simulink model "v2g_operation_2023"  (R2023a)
settings: Solver=VariableStepAuto  StartTime=0.0  StopTime=0.1  FixedStep=1e-7  MaxStep=1e-5  RelTol=1e-3
libraries: spsMosfetLib x4, spsCurrentMeasurementLib x2, spsACVoltageSourceLib x1, spsPowerLib x1, spsVoltageMeasurementLib x1, spsDCVoltageSourceLib x1, spsSeriesRLCBranchLib x1, simulink x1, spspowerguiLib x1

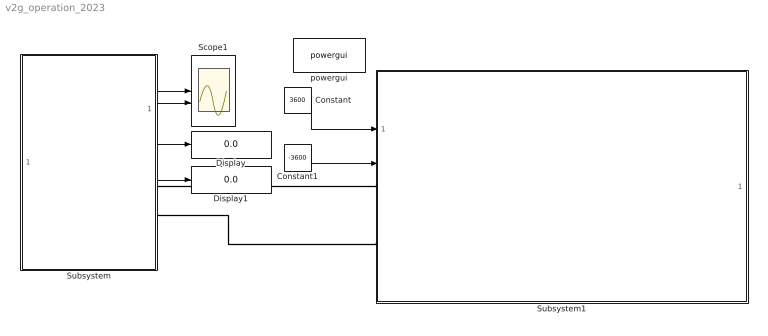
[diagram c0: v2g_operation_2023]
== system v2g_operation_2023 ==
  Constant : Constant  Value=3600
  Constant1 : Constant  Value=-3600
  Display : Display
  Display1 : Display
  Scope1 : Scope  NumInputPorts=2
  Subsystem : Subsystem
  Subsystem1 : Subsystem
  powergui : spspowerguiLib/powergui  Priority=1  SimulationMode=Continuous  SampleTime=50e-6  frequency=60  Iterations=50  frequencyindice=60  Pbase=100e6  ErrMax=1e-4  UnitsV=kV  UnitsW=MW  buscounter=0  FunctionMessages=off  echomessages=off  EnableUseOfTLC=off  CurrentSourceSwitches=off  DisableSnubberDevices=off  DisableRonSwitches=off  DisableVfSwitches=off  DisplayEquations=off  AutomaticDiscreteSolvers=off  SolverType=Tustin/Backward Euler (TBE)  Interpol=off  ExternalGateDelay=off  methode=off  Ts=100  x0status=blocks  SPID=on  SwTol=0  HookPort=off  NonlinearTolerance=1e-4  nMaxIteration=100  ContinueOnMaxIteration=off  RestoreLinks=warning  ResistiveCurrentMeasurement=off  Frange=[0:2:500]  Ylog=off  Xlog=on  ShowGrid=off  save=off  variable=ZData  structure=0  ZoomFFT=off  StartTime=0.0  cycles=1  DisplayStyle=1  fundamental=60  FreqAxis=off  MaxFrequency=1000  frequencyindicesteady=1  RmsSteady=1  display=off
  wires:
  Subsystem/1(vac) -> Scope1/1
  Subsystem/2(iac) -> Scope1/2
  Subsystem/3(P) -> Display/1
  Subsystem/4(Q) -> Display1/1
  Constant/1 -> Subsystem1/1(Pref)
  Constant1/1 -> Subsystem1/2(Qref)
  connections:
  Subsystem/RConn1 -- Subsystem1/LConn1
  Subsystem/RConn2 -- Subsystem1/LConn2

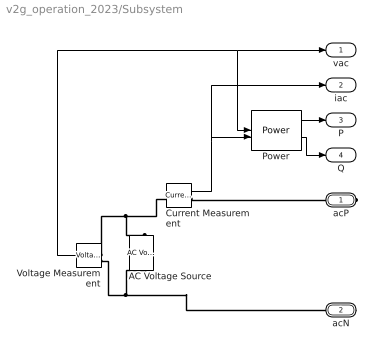
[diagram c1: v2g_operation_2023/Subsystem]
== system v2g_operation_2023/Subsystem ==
  AC Voltage Source : spsACVoltageSourceLib/AC Voltage Source  Amplitude=220*sqrt(2)  Phase=0  Frequency=60  SampleTime=0  Measurements=None  BusType=swing  Pref=10e3  Qref=0  Qmin=-inf  Qmax=+inf
  Current Measurement : spsCurrentMeasurementLib/Current Measurement  PhasorSimulation=off  OutputType=Complex  PSBequivalent=0
  Power : spsPowerLib/Power  Freq=60  Vinit=[1, 0]  Iinit=[1, 0]  Ts=0
  Voltage Measurement : spsVoltageMeasurementLib/Voltage Measurement  PhasorSimulation=off  OutputType=Complex  PSBequivalent=0
  acP : PMIOPort  Side=Right
  acN : PMIOPort  Port=2  Side=Right
  vac : Outport
  iac : Outport  Port=2
  P : Outport  Port=3
  Q : Outport  Port=4
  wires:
  Voltage Measurement/1 -> Power/1, vac/1
  Current Measurement/1 -> Power/2, iac/1
  Power/1 -> P/1
  Power/2 -> Q/1
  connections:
  Voltage Measurement/LConn2 -- acN/RConn1 -- AC Voltage Source/LConn1
  Voltage Measurement/LConn1 -- AC Voltage Source/RConn1 -- Current Measurement/LConn1
  Current Measurement/RConn1 -- acP/RConn1

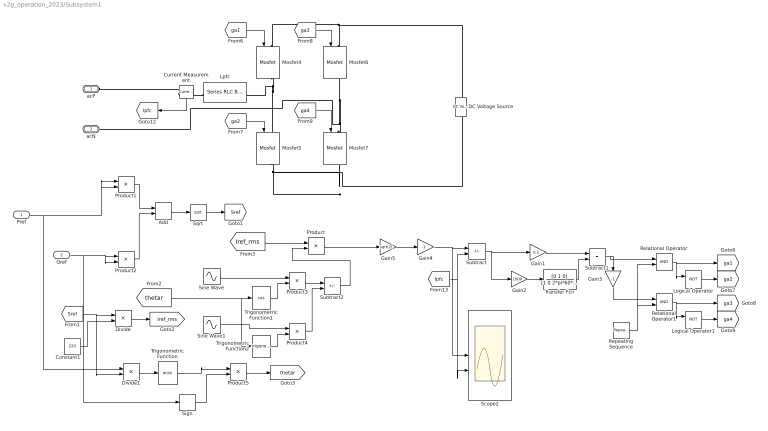
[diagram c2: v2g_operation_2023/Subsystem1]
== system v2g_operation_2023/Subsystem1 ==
  Pref : Inport
  Qref : Inport  Port=2
  Add : Sum
  Constant1 : Constant  Value=220
  Current Measurement : spsCurrentMeasurementLib/Current Measurement  PhasorSimulation=off  OutputType=Complex  PSBequivalent=0
  DC Voltage Source : spsDCVoltageSourceLib/DC Voltage Source  Amplitude=380  Measurements=None
  Divide : Product  Inputs=*/
  Divide1 : Product  Inputs=*/
  Gain1 : Gain  Gain=0.1
  Gain2 : Gain  Gain=1000
  Gain3 : Gain  Gain=-1
  Gain4 : Gain  Gain=-1
  Gain5 : Gain  Gain=sqrt(2)
  Logical Operator : Logic  Operator=NOT  AllPortsSameDT=off  OutDataTypeStr=boolean
  Logical Operator1 : Logic  Operator=NOT  AllPortsSameDT=off  OutDataTypeStr=boolean
  Lpfc : spsSeriesRLCBranchLib/Series RLC Branch  LConnTagsString=__new0  RConnTagsString=__new0  BranchType=L  Resistance=20  Inductance=5e-3  SetiL0=off  InitialCurrent=0  Capacitance=3e-3  Setx0=on  InitialVoltage=380  Measurements=Branch current
  Mosfet{4..7} (4 alike) : spsMosfetLib/Mosfet  Ron=0.1  Lon=0  Rd=0.01  Vfd=0  IC=0  Rs=1e5  Cs=inf  Measurements=on
  Product{,1..5} (6 alike) : Product
  Relational Operator : RelationalOperator  OutDataTypeStr=boolean  RndMeth=Simplest
  Relational Operator1 : RelationalOperator  OutDataTypeStr=boolean  RndMeth=Simplest
  Repeating Sequence : simulink/Sources/Repeating Sequence  rep_seq_t=[0 0.00005]  rep_seq_y=[0 1]
  Scope2 : Scope  NumInputPorts=2
  Sign : Signum
  Sine Wave : Sin  Frequency=2*pi*60  SampleTime=0
  Sine Wave1 : Sin  Frequency=2*pi*60  Phase=pi/2  SampleTime=0
  Sqrt : Sqrt
  Subtract : Sum  Inputs=+-
  Subtract1 : Sum
  Subtract2 : Sum  Inputs=+-
  Transfer Fcn : TransferFcn  Numerator=[0 1 0]  Denominator=[1 0 2*pi*60*2*pi*60]
  Trigonometric Function : Trigonometry  Operator=acos
  Trigonometric Function1 : Trigonometry  Operator=cos
  Trigonometric Function2 : Trigonometry
  acP : PMIOPort  Side=Left
  acN : PMIOPort  Port=2  Side=Left
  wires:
  Repeating Sequence/1 -> Relational Operator1/2, Relational Operator/2
  [ga2] -> Mosfet5/1
  [ga4] -> Mosfet7/1
  Subtract1/1 -> Gain3/1, Relational Operator/1
  Gain1/1 -> Subtract1/1
  [ga3] -> Mosfet6/1
  Product/1 -> Gain5/1
  [Ipfc] -> Subtract/2, Scope2/2
  Relational Operator/1 -> [ga1], Logical Operator/1
  Subtract/1 -> Gain2/1, Gain1/1
  Relational Operator1/1 -> [ga3], Logical Operator1/1
  Gain3/1 -> Relational Operator1/1
  Gain2/1 -> Transfer Fcn/1
  Transfer Fcn/1 -> Subtract1/2
  Current Measurement/1 -> [Ipfc]
  Logical Operator1/1 -> [ga4]
  Logical Operator/1 -> [ga2]
  [ga1] -> Mosfet4/1
  Pref/1 -> Divide1/1, Product1/2, Product1/1
  Product1/1 -> Add/1
  Product2/1 -> Add/2
  Add/1 -> Sqrt/1
  Sqrt/1 -> [Sref]
  [Sref] -> Divide1/2, Divide/1
  Constant1/1 -> Divide/2
  Divide/1 -> [Iref_rms]
  Divide1/1 -> Trigonometric Function/1
  Gain4/1 -> Scope2/1, Subtract/1
  Sine Wave/1 -> Product3/1
  Trigonometric Function1/1 -> Product3/2
  [thetar] -> Trigonometric Function2/1, Trigonometric Function1/1
  Sine Wave1/1 -> Product4/1
  Trigonometric Function2/1 -> Product4/2
  Product3/1 -> Subtract2/1
  Product4/1 -> Subtract2/2
  Subtract2/1 -> Product/2
  [Iref_rms] -> Product/1
  Gain5/1 -> Gain4/1
  Qref/1 -> Product2/2, Product2/1, Sign/1
  Product5/1 -> [thetar]
  Trigonometric Function/1 -> Product5/1
  Sign/1 -> Product5/2
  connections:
  Mosfet4/RConn1 -- Mosfet5/LConn1 -- Lpfc/LConn1
  Mosfet7/LConn1 -- acN/RConn1 -- Mosfet6/RConn1
  Mosfet4/LConn1 -- DC Voltage Source/RConn1 -- Mosfet6/LConn1
  Mosfet5/RConn1 -- DC Voltage Source/LConn1 -- Mosfet7/RConn1
  Current Measurement/LConn1 -- Lpfc/RConn1
  Current Measurement/RConn1 -- acP/RConn1
